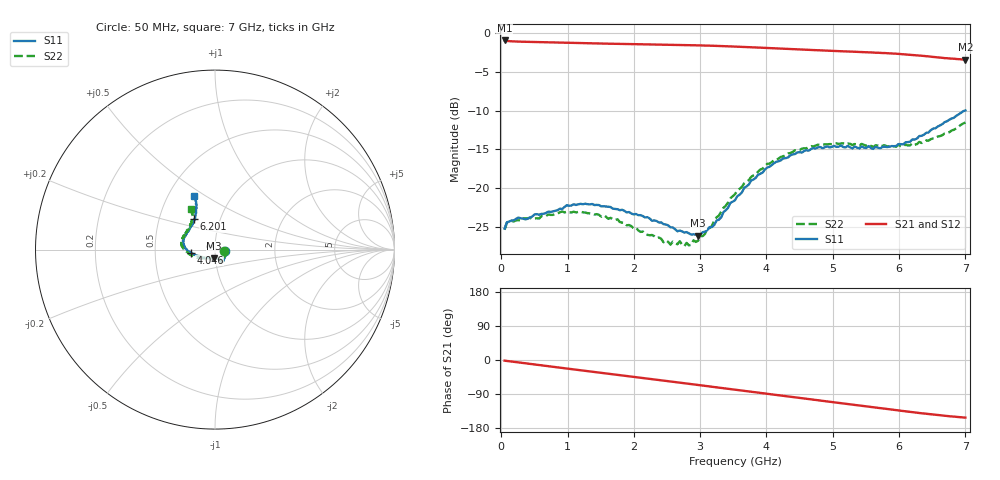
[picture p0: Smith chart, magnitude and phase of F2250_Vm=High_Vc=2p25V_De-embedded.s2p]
! Integrated Device Technology
! Corporate Headquarters
! 6024 Silver Creek Valley Road
! San Jose, CA 95138  USA
! Phone:  1-408-284-8200
! Toll Free:  1-800-223-1366
! Webpage:  http://www.idt.com/
! Timing and RF Division
! 515 Groton Road, Suite 102
! Westford, MA 01886-6024
! Device:  F2250
! Description: Voltage Variable RF Attenuator
! Frequency:  50.0 -  6000.00 MHz
! Package:  3x3 mm Thin QFN Plastic Package: 16 pin
! Ports:  2 RF, 3 DC
!  Pin  1  = GND
!  Pin  2  = NC
!  Pin  3  = RF1  = Port 1
!  Pin  4  = NC
!  Pin  5  = GND
!  Pin  6  = GND
!  Pin  7  = GND
!  Pin  8  = GND
!  Pin  9  = NC
!  Pin 10  = RF2  = Port 2
!  Pin 11  = NC
!  Pin 12  = GND
!  Pin 13  = GND
!  Pin 14  = VCNTRL
!  Pin 15  = VDD
!  Pin 16  = VMODE
! Vcntrl:  2.250 Volts
! Vmode:  +3.300 Volts
! Vdd:  +3.30  Volts
! Current:  1.316 mA
! Data:  The device was measured on a the F2250 evaluation board which has
!  individual transmission lines to the RF pins.  Data was collected
!  using a calibrated network analyzer.  The evaluation board was
!  de-embedded using a TRL calibration technique.
!  The reference plane is the edge of the package pin.
! Misc:  SN 10
!  Action Tracker AT0258
! Date Measured:  2014-11-26
! Date:  2015-10-15  MJV
! Note:
!  Integrated Device Technology supplies this data as a sample of measured
!  data at the package pin for this product.  Your particular data for this
!  product may vary.
!  Data was taken at 25 degrees C.
!  Integrated Device Technology reserves the right to change this data at anytime.
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# GHz S dB R 50
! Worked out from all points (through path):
!   201 points, 50 MHz to 7 GHz, reference 50 ohm
!   highest |S21| = -0.92 dB at 50 MHz (marker M1); lowest = -3.4 dB at 7 GHz (marker M2)
!   group delay of S21, straight-line fit = 61.1 ps
!   lowest |S11| = -26.1 dB at 2.969 GHz (marker M3), VSWR 1.10, Z = 49.3 - j4.85 ohm
!   |S11| at or under -10 dB: start of sweep to 6.99 GHz
!   |S22| runs from -27.5 to -11.5 dB; largest |S21 - S12| = 0.0019
!   S11 on the Smith chart (normalised r, x): 50 MHz: 1.11, -0.02; 4.046 GHz: 0.76, -0.03; 6.201 GHz: 0.75, +0.27; 7 GHz: 0.68, +0.45
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0.05  -25.23 -10.1  -0.92 -1.8  -0.92 -1.8  -25.40 -10.5
0.1195  -24.32 -9.8  -1.01 -3.2  -1.01 -3.2  -24.29 -8.7
0.91875  -22.70 -48.7  -1.20 -21.0  -1.20 -21.1  -23.03 -50.2
1.2315  -22.09 -56.5  -1.27 -27.9  -1.27 -27.9  -23.15 -60.7
1.75275  -22.74 -63.4  -1.36 -39.1  -1.36 -39.1  -24.04 -67.4
2.37825  -24.46 -63.3  -1.45 -52.8  -1.45 -52.8  -26.39 -67.5
2.552  -25.08 -68.0  -1.47 -56.6  -1.47 -56.7  -27.32 -73.9
2.691  -25.50 -75.8  -1.50 -59.8  -1.50 -59.8  -26.88 -81.5
2.7605  -25.75 -77.9  -1.51 -61.3  -1.51 -61.3  -27.52 -85.9
2.969  -26.15 -95.3  -1.55 -66.0  -1.55 -66.0  -26.81 -104.8
3.21225  -24.77 -125.2  -1.61 -71.5  -1.61 -71.5  -24.18 -129.6
3.4555  -21.91 -146.4  -1.68 -76.9  -1.68 -77.0  -21.31 -144.9
3.525  -21.58 -150.8  -1.71 -78.5  -1.71 -78.6  -20.79 -148.2
3.76825  -19.03 -163.3  -1.80 -84.0  -1.80 -84.0  -18.57 -159.2
4.04625  -17.25 -172.9  -1.91 -90.2  -1.91 -90.2  -16.84 -169.6
4.4285  -15.61 176.9  -2.06 -98.6  -2.06 -98.6  -15.13 179.0
4.7065  -14.83 169.9  -2.16 -104.8  -2.16 -104.8  -14.62 173.2
5.054  -14.68 161.7  -2.29 -112.5  -2.28 -112.5  -14.22 166.1
5.85325  -14.66 135.7  -2.58 -130.0  -2.58 -130.1  -14.63 147.4
6.20075  -13.71 124.1  -2.79 -137.7  -2.79 -137.8  -14.21 138.3
6.54825  -12.26 116.0  -3.06 -144.7  -3.07 -144.8  -13.55 127.0
7  -9.97 111.1  -3.39 -152.1  -3.40 -152.2  -11.53 120.7
